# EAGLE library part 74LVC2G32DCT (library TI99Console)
2-input OR gate
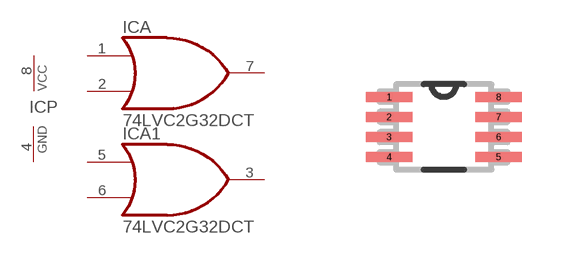
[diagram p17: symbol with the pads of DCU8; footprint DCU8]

Designator prefix IC; gates A=7432 P=PWRN A1=7432

## 74LVC2G32DCT  [DCU8]
1  A:I0  in
2  A:I1  in
3  A1:O  out
4  P:GND  pwr
5  A1:I0  in
6  A1:I1  in
7  A:O  out
8  P:VCC  pwr

## Footprint DCU8 (pad centres in mm)
smd 1.168 x 0.254: 1 -1.372,0.75; 2 -1.372,0.25; 3 -1.372,-0.25; 4 -1.372,-0.75; 5 1.372,-0.75; 6 1.372,-0.25; 7 1.372,0.25; 8 1.372,0.75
